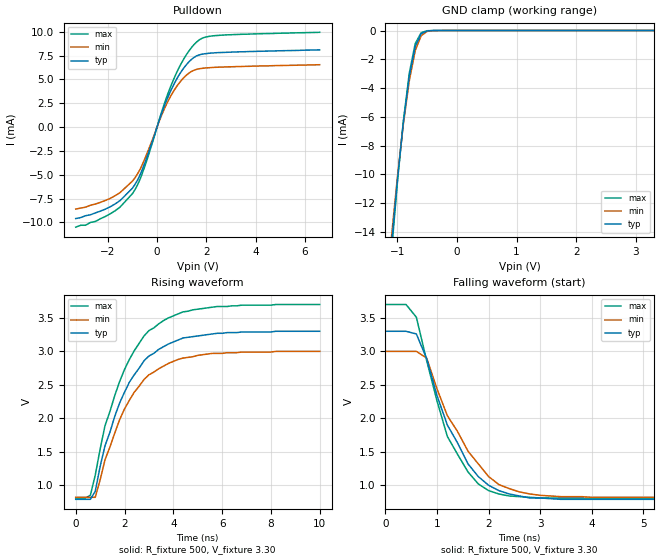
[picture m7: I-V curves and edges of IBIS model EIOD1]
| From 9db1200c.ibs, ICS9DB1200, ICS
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|   Model EIOD1
[Model]   EIOD1
Model_type   I/O_open_drain
Polarity   Inverting
Enable   Active-High
Vinl =   0.80V
Vinh =   2.00V
Vmeas =   1.50V
Cref =  30.00pF
Rref =  2700.000
Vref =   1.50V
C_comp   5.50pF   5.00pF   6.00pF
[Temperature Range]   27.00   70.00   0.000
[Voltage Range]   3.30V   3.00V   3.70V
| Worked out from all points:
|   slope of the pulldown table from 0 to 0.495 V, typ, clamps not added: 143 ohm
|   GND clamp passes 1 mA (typ) near -0.69 V on its own axis
|   rising waveform, R_fixture 500, V_fixture 3.30: 20-80 % time 1.68ns typ, 1.65ns min, 1.68ns max; typ from 0.79 V to 3.3 V
|   falling waveform, R_fixture 500, V_fixture 3.30: 20-80 % time 796ps typ, 921ps min, 736ps max; typ from 3.3 V to 0.79 V
[Pulldown]
| voltage   I(typ)   I(min)   I(max)
-3.3V     -9.6mA     -8.6mA     -10.5mA
-2.5V     -9mA       -8.07mA    -9.9mA
-1.9V     -8.36mA    -7.48mA    -9.1mA
-1.5V     -7.71mA    -6.87mA    -8.39mA
-1V       -6.41mA    -5.67mA    -6.99mA
-600mV    -4.47mA    -3.95mA    -4.87mA
200mV     1.54mA     1.34mA     1.71mA
700mV     4.58mA     3.89mA     5.18mA
1.2V      6.58mA     5.47mA     7.64mA
1.7V      7.57mA     6.12mA     9.13mA
2.6V      7.83mA     6.3mA      9.65mA
6.6V      8.11mA     6.55mA     9.95mA
[GND_clamp]
| voltage   I(typ)   I(min)   I(max)
-3.3V     -140mA     -130mA     -150mA
-1.1V     -15.03mA   -14.42mA   -15.5mA
-1V       -10.44mA   -10.24mA   -10.61mA
-900mV    -6.42mA    -6.54mA    -6.34mA
-800mV    -3.2mA     -3.51mA    -2.98mA
-700mV    -1.11mA    -1.4mA     -910uA
-600mV    -220uA     -360uA     -150uA
-500mV    -27.68uA   -59.47uA   -15.28uA
-400mV    -2.43uA    -7.38uA    -1.01uA
3.3V      150pA      520pA      120pA
[Ramp]
| variable   typ   min   max
dV/dt_r   1.50/1.65n   1.31/1.63n   1.74/1.64n
dV/dt_f   1.51/0.74n   1.31/0.87n   1.74/0.67n
R_load = 500
[Rising Waveform]
R_fixture = 500
V_fixture = 3.30
V_fixture_min = 3.00
V_fixture_max = 3.70
| time   V(typ)   V(min)   V(max)
0s        790mV      820mV      810mV
600ps     790mV      820mV      850mV
800ps     910mV      820mV      1.15V
1.2ns     1.59V      1.38V      1.89V
1.8ns     2.23V      1.98V      2.55V
2.4ns     2.65V      2.39V      3.01V
3ns       2.93V      2.65V      3.31V
3.8ns     3.11V      2.82V      3.5V
4.8ns     3.22V      2.92V      3.62V
10ns      3.3V       3V         3.7V
[Falling Waveform]
R_fixture = 500
V_fixture = 3.30
V_fixture_min = 3.00
V_fixture_max = 3.70
| time   V(typ)   V(min)   V(max)
0s        3.3V       3V         3.7V
400ps     3.3V       3V         3.7V
600ps     3.26V      3V         3.51V
800ps     2.89V      2.9V       2.86V
1.2ns     1.9V       2.04V      1.73V
1.6ns     1.32V      1.51V      1.2V
2ns       1V         1.13V      920mV
2.6ns     840mV      900mV      830mV
3.4ns     790mV      830mV      810mV
10ns      790mV      820mV      810mV
